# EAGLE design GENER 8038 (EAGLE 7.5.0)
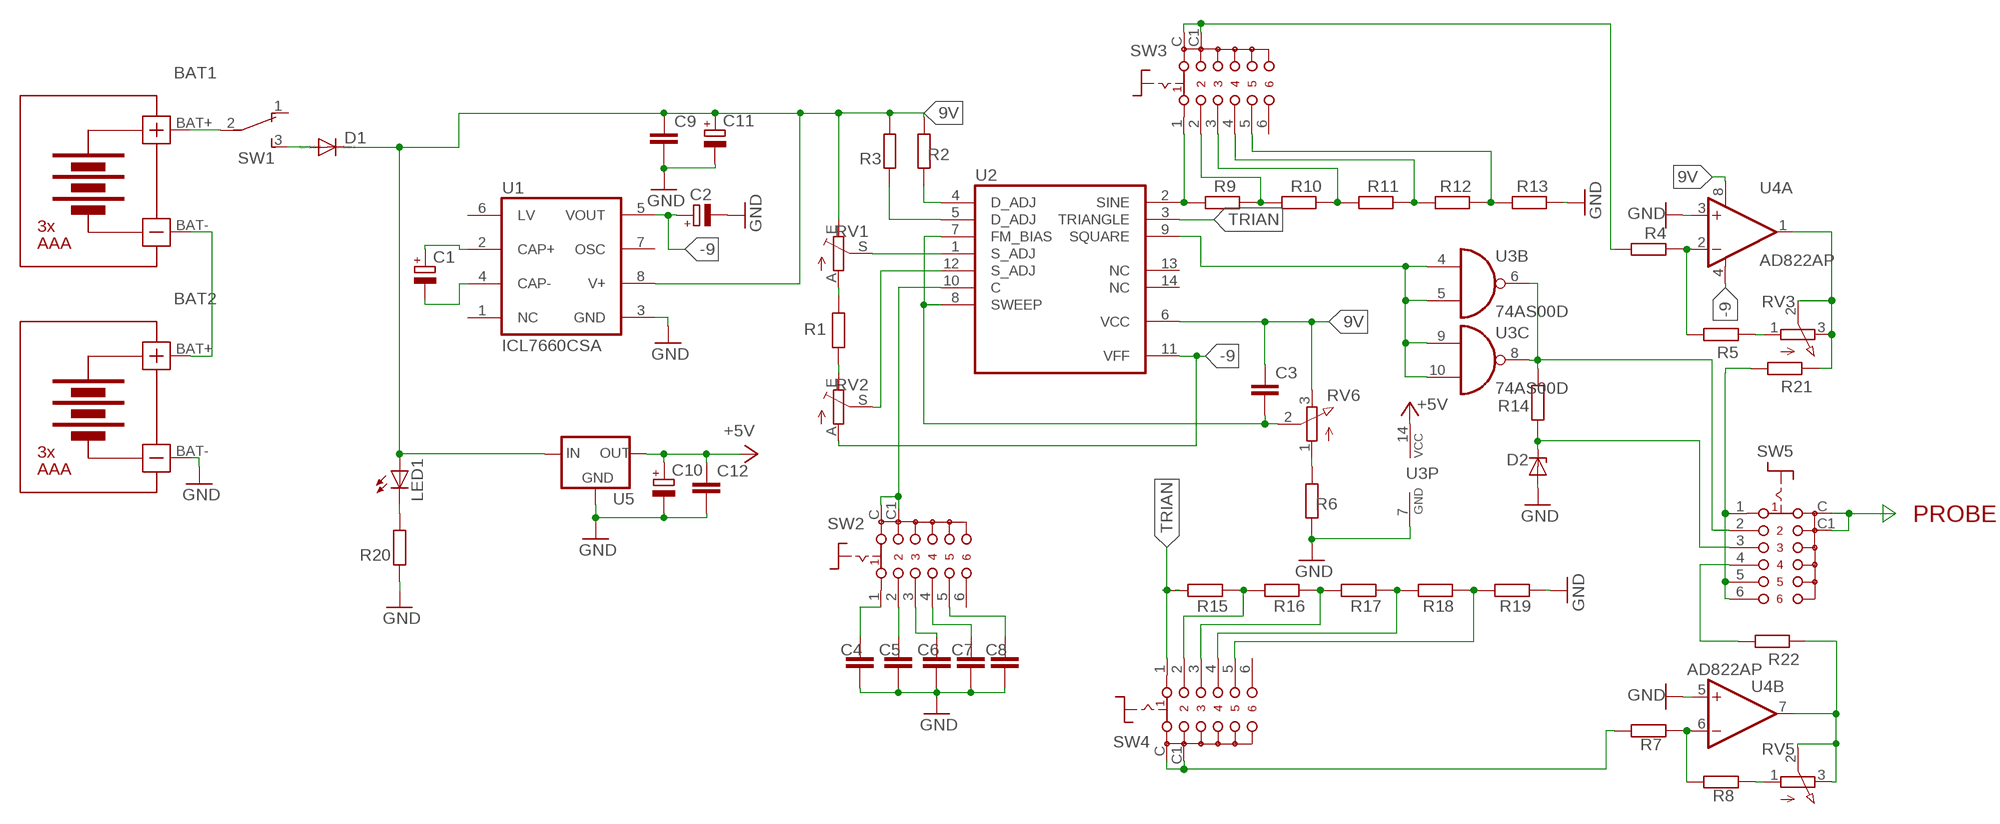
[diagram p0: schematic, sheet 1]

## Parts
BAT1  BATTERY-HOLDER-3AAA  [BATTERY-HOLDER-3AAA]
BAT2  BATTERY-HOLDER-3AAA  [BATTERY-HOLDER-3AAA]
C1  CPOL-EUC/6032-28W  [C/6032-28W]
C2  CPOL-EUC/6032-28W  [C/6032-28W]
C3  C-EUC1206  [C1206]
C4  C-EUC1206  [C1206]
C5  C-EUC1206  [C1206]
C6  C-EUC1206  [C1206]
C7  C-EUC1206  [C1206]
C8  C-EUC1206  [C1206]
C9  C-EUC1206  [C1206]
C10  CPOL-EUC/6032-28W  [C/6032-28W]
C11  CPOL-EUC/6032-28W  [C/6032-28W]
C12  C-EUC1206  [C1206]
D1  1N4148DO35-7  [DO35-7]
D2  BZX85  [DO41Z10]
LED1  LED3MM  [LED3MM]
R1  R-EU_R1206  [R1206]
R2  R-EU_R1206  [R1206]
R3  R-EU_R1206  [R1206]
R4  R-EU_R1206  [R1206]
R5  R-EU_R1206  [R1206]
R6  R-EU_R1206  [R1206]
R7  R-EU_R1206  [R1206]
R8  R-EU_R1206  [R1206]
R9  R-EU_R1206  [R1206]
R10  R-EU_R1206  [R1206]
R11  R-EU_R1206  [R1206]
R12  R-EU_R1206  [R1206]
R13  R-EU_R1206  [R1206]
R14  R-EU_R1206  [R1206]
R15  R-EU_R1206  [R1206]
R16  R-EU_R1206  [R1206]
R17  R-EU_R1206  [R1206]
R18  R-EU_R1206  [R1206]
R19  R-EU_R1206  [R1206]
R20  R-EU_R1206  [R1206]
R21  R-EU_R1206  [R1206]
R22  R-EU_R1206  [R1206]
RV1  TRIM_EU-CT6  [CT6]
RV2  TRIM_EU-CT6  [CT6]
RV3  PTV09A  PV09A  [PTV09]
RV5  PTV09A  PV09A  [PTV09]
RV6  PTV09A  PV09A  [PTV09]
SW1  TL36YO  [TL3XYO]
SW2  SS-10-16  [SS-10-16]
SW3  SS-10-16  [SS-10-16]
SW4  SS-10-16  [SS-10-16]
SW5  SS-10-16  [SS-10-16]
U1  ICL7660CSA  [SO08]
U2  XR-8038  [DIL14]
U3  74AS00D  [SO14]
U4  AD822AP  OPA2131U  [SO08]
U5  78LXX  [78LXX]

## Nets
9V: C3.1 C9.1 C11.+ D1.C LED1.A R2.2 R3.2 RV1.E RV6.3(E) U1.8(V+) U2.6(VCC) U4.8(A:V+) U5.IN
+5V: C10.+ C12.1 U3.14(P:VCC) U5.OUT
-9: C2.+ RV2.A U1.5(VOUT) U2.11(VFF) U4.4(A:V-)
GND: BAT2.BAT- C2.- C4.2 C5.2 C6.2 C7.2 C8.2 C9.2 C10.- C11.- C12.2 D2.A R6.1 R13.1 R19.1 R20.1 U1.3(GND) U3.7(P:GND) U4.3(A:+IN) U4.5(B:+IN) U5.GND
N$1: BAT1.BAT- BAT2.BAT+
N$2: BAT1.BAT+ SW1.2(P)
N$3: R2.1 U2.4(D_ADJ)
N$4: R3.1 U2.5(D_ADJ)
N$5: RV1.S U2.1(S_ADJ)
N$6: R1.2 RV1.A
N$7: R1.1 RV2.E
N$8: RV2.S U2.12(S_ADJ)
N$9: C3.2 RV6.2(S) U2.7(FM_BIAS) U2.8(SWEEP)
N$10: SW2.C SW2.C1 U2.10(C)
N$11: R6.2 RV6.1(A)
N$12: C4.1 SW2.1
N$13: C5.1 SW2.2
N$14: C6.1 SW2.3
N$15: C7.1 SW2.4
N$16: C8.1 SW2.5
N$17: R9.2 SW3.1 U2.2(SINE)
N$18: R9.1 R10.2 SW3.2
N$19: R10.1 R11.2 SW3.3
N$20: R11.1 R12.2 SW3.4
N$21: R12.1 R13.2 SW3.5
N$22: U2.9(SQUARE) U3.4(B:I0) U3.5(B:I1) U3.9(C:I0) U3.10(C:I1)
N$23: R15.1 R16.2 SW4.2
N$24: R16.1 R17.2 SW4.3
N$25: R17.1 R18.2 SW4.4
N$26: R18.1 R19.2 SW4.5
N$27: R14.2 SW5.2 U3.6(B:O) U3.8(C:O)
N$28: D2.C R14.1 SW5.3
N$29: R21.2 SW5.1 SW5.5 SW5.6
N$30: R4.1 R5.2 U4.2(A:-IN)
N$31: R5.1 RV3.1(A)
N$32: R4.2 SW3.C SW3.C1
N$33: R7.1 R8.2 U4.6(B:-IN)
N$34: R8.1 RV5.1(A)
N$35: R22.1 RV5.2(S) RV5.3(E) U4.7(B:OUT)
N$36: R7.2 SW4.C SW4.C1
N$37: SW5.C SW5.C1
N$38: D1.A SW1.3(S)
N$39: LED1.K(C) R20.2
N$40: R21.1 RV3.2(S) RV3.3(E) U4.1(A:OUT)
N$41: R22.2 SW5.4
N$84: C1.+ U1.2(CAP+)
N$85: C1.- U1.4(CAP-)
TRIAN: R15.2 SW4.1 U2.3(TRIANGLE)
Unconnected: SW1.1(O) SW2.6 SW3.6 SW4.6 U1.1(NC) U1.6(LV) U1.7(OSC) U2.13(NC) U2.14(NC) U3.1(A:I0) U3.2(A:I1) U3.3(A:O) U3.11(D:O) U3.12(D:I0) U3.13(D:I1)

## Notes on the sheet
- PROBE

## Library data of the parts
BAT1 BAT2 = diy-modules:BATTERY-HOLDER-3AAA
C1 C2 C10 C11 = rcl:CPOL-EU: POLARIZED CAPACITOR, European symbol
C3-C9 C12 = rcl:C-EU: CAPACITOR, European symbol
D1 = diode:1N4148: DIODE
D2 = diode:BZX85: Z DIODE
LED1 = led:LED: LED
R1-R22 = rcl:R-EU_: RESISTOR, European symbol
RV1 RV2 = pot:TRIM_EU-: POTENTIOMETER
RV3 RV5 RV6 = pot:PV09A
SW1 = switch:TL36YO: TINY SWITCH ON - ON Source: http://www2.produktinfo.conrad.com/datenblaetter/700000-724999/705152-da-01-de-Subminiaturschalter_TL_36YO.pdf
SW2-SW5 = switch:SS-10-16: Rotary Switch, Through Hole, 6 Position, 1 Pole
U1 = maxim:ICL7660CSA: VOLTAGE CONVERTER; MF: MAXIM; MPN: ICL7660CSA; OC_FARNELL: 9724710; OC_NEWARK: 34C3732
U2 = exar:XR-8038: Precision WAVEFORM GENERATOR; OC_FARNELL: unknown; OC_NEWARK: unknown
U3 = 74xx-eu:74*00: Quad 2-input NAND gate
U4 = burr-brown:OPA2131: General Purpose FET-Input Operational Amplifiers Product Folder:OPA2131; MF: TEXAS INSTRUMENT CONNECTORS; MPN: OPA2131UJ/2K5; OC_FARNELL: 1575488; OC_NEWARK: 75C4620
U5 = v-reg:78LXX: VOLTAGE REGULATOR

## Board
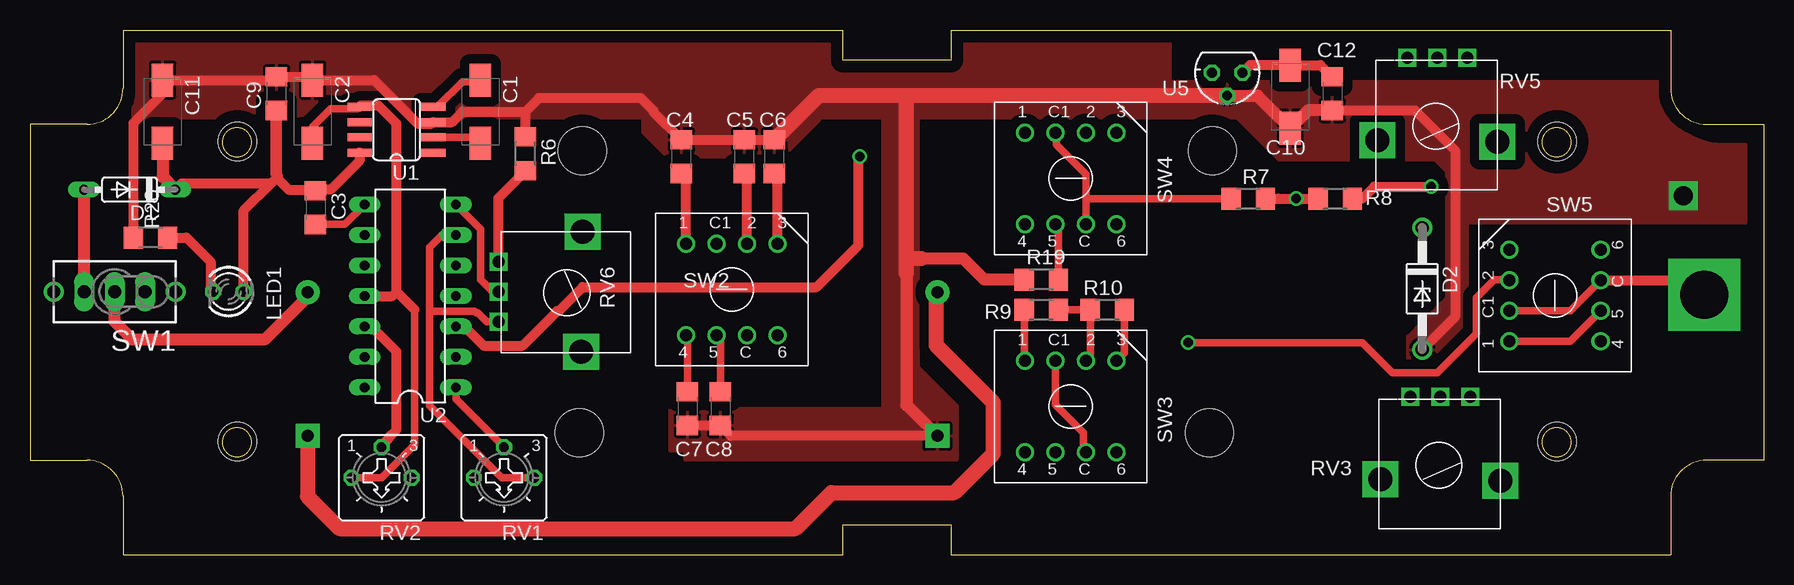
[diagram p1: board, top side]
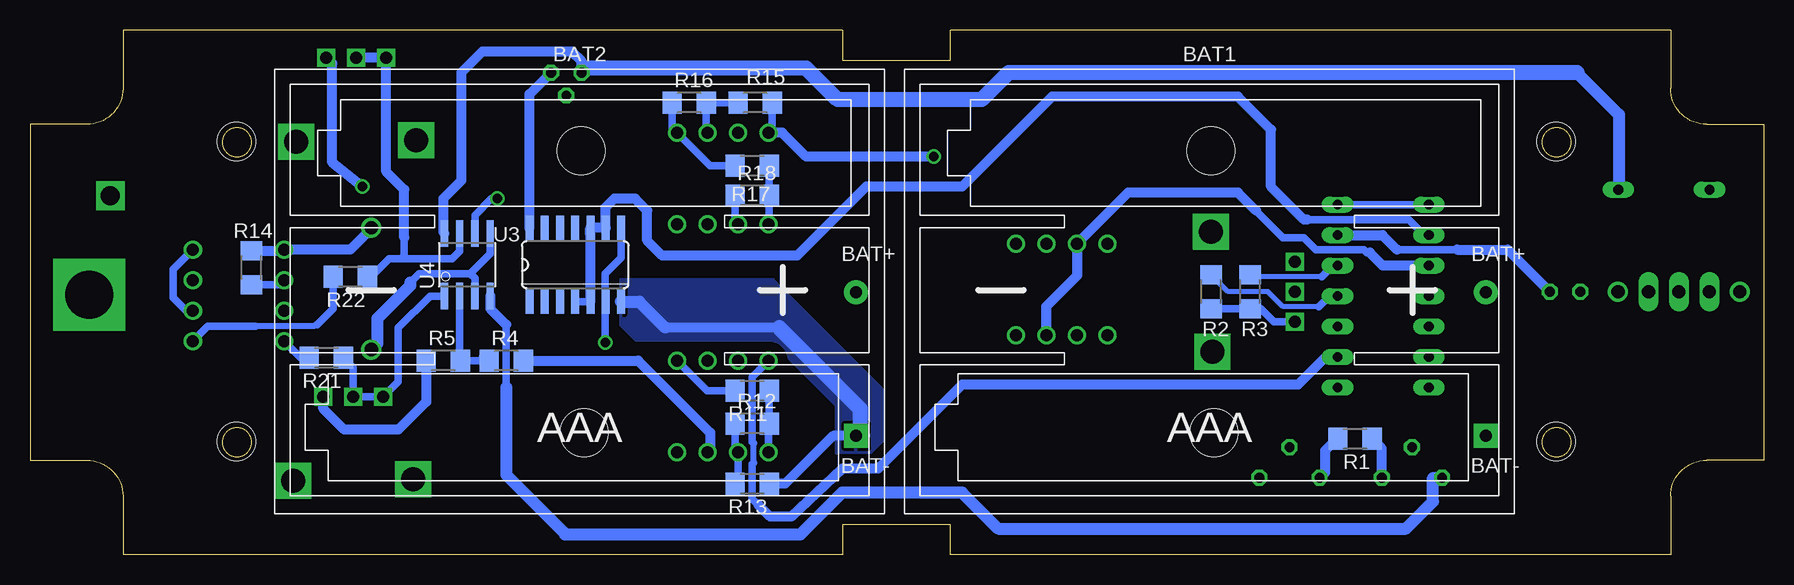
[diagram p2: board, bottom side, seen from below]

Size 144.5 x 43.72 mm. Coordinates in mm from the lower left corner, seen from the top.
Outline: 76.75,41.22 67.75,41.22 67.75,43.72 7.75,43.72 7.75,38.86 arc-90 4.75,35.86 0,35.86 0,7.86 4.75,7.86 arc-90 7.75,4.86 7.75,0 67.75,0 67.75,2.5 76.75,2.5 76.75,0 136.75,0 136.75,4.86 arc-90 139.75,7.86 144.5,7.86 144.5,35.86 139.75,35.86 arc-90 136.75,38.86 136.75,43.72 76.75,43.72 76.75,41.22
Outline: circle at 17.25,34.36 radius 1.2
Outline: circle at 17.25,9.36 radius 1.2
Outline: circle at 127.25,34.36 radius 1.2
Outline: circle at 127.25,9.36 radius 1.2
Copper layers (1*16): Top 0.035mm / dielectric 1.5mm / Bottom 0.035mm
Design rules "default": minimum track width 10mil, minimum drill 24mil, track to track 8mil, track to pad 8mil, pad to pad 8mil, via to via 8mil, smd to smd 8mil, copper to edge 40mil, drill to drill 8mil, minimum pad ring 10mil, minimum via ring 8mil, stop-mask expansion 4mil, vias tented up to drill 0mil, thermal gap 10mil
Holes 3.2 mm at 17.3,34.41 17.3,9.41 127.3,34.41 127.3,9.41

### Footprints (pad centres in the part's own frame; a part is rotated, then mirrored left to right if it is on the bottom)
BATTERY-HOLDER-3AAA = drill 1 pad 2: BAT+ 22.425,0.46 | drill 1 pad 2 square: BAT- 22.425,-11.51 | hole 4: -0.5,12.25; -0.25,-11.25
C/6032-28W = smd 2.75 x 1.8: + 2.625,0; - -2.625,0
C1206 = smd 1.6 x 1.8: 1 -1.4,0; 2 1.4,0
DO35-7 = drill 0.813 long: A 3.81,0; C -3.81,0
DO41Z10 = drill 1.118: A 5.08,0; C -5.08,0
LED3MM = drill 0.813 octagon: A -1.27,0; K 1.27,0
R1206 = smd 1.6 x 1.803: 1 -1.422,0; 2 1.422,0
CT6 = drill 0.813 octagon: A 2.515,0; E -2.515,0; S 0,-2.54
PTV09 = drill 1 square: 1 -2.5,0; 2 0,0; 3 2.5,0 | drill 2 square: P$4 -5,7; P$5 5,6.9
TL3XYO = drill 1.1 pad 1.422 long: 1 -2.54,0; 2 0,0; 3 2.54,0 | drill 1.1 pad 1.676: M1 -5.08,0; M2 5.08,0
SS-10-16 = drill 1: 1 -7.62,0; 2 -2.54,0; 3 0,0; 4 -7.62,-7.62; 5 -5.08,-7.62; 6 0,-7.62; C -2.54,-7.62; C1 -5.08,0
SO08 = smd 0.66 x 2.032: 1 -1.905,-3.073; 2 -0.635,-3.073; 3 0.635,-3.073; 4 1.905,-3.073; 5 1.905,3.073; 6 0.635,3.073; 7 -0.635,3.073; 8 -1.905,3.073
DIL14 = drill 0.813 long: 1 -7.62,-3.81; 2 -5.08,-3.81; 3 -2.54,-3.81; 4 0,-3.81; 5 2.54,-3.81; 6 5.08,-3.81; 7 7.62,-3.81; 8 7.62,3.81; 9 5.08,3.81; 10 2.54,3.81; 11 0,3.81; 12 -2.54,3.81; 13 -5.08,3.81; 14 -7.62,3.81
SO14 = smd 0.66 x 2.032: 1 -3.81,-3.073; 2 -2.54,-3.073; 3 -1.27,-3.073; 4 0,-3.073; 5 1.27,-3.073; 6 2.54,-3.073; 7 3.81,-3.073; 8 3.81,3.073; 9 2.54,3.073; 10 1.27,3.073; 11 0,3.073; 12 -1.27,3.073; 13 -2.54,3.073; 14 -3.81,3.073
SO08' = smd 0.61 x 2.21: 1 -1.905,-2.616; 2 -0.635,-2.616; 3 0.635,-2.616; 4 1.905,-2.616; 5 1.905,2.616; 6 0.635,2.616; 7 -0.635,2.616; 8 -1.905,2.616
78LXX = drill 0.813 octagon: GND 0,1.905; IN 1.27,0; OUT -1.27,0

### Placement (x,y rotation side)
BAT1  45.55,21.41 0 bottom
BAT2  98.05,21.41 0 bottom
C1  37.55,36.91 270 top
C2  23.55,36.91 270 top
C3  23.8,28.91 270 top
C4  54.3,33.16 90 top
C5  59.55,33.16 90 top
C6  62.05,33.16 90 top
C7  54.8,12.16 270 top
C8  57.55,12.16 270 top
C9  20.55,38.41 90 top
C10  105.05,38.16 90 top
C11  11.05,36.91 270 top
C12  108.55,38.41 270 top
D1  8.3,30.41 180 top
D2  116.05,22.16 270 top
LED1  16.55,21.91 180 top
R1  34.05,9.66 180 bottom
R2  46.05,21.91 270 bottom
R3  42.8,21.91 270 bottom
R4  104.8,16.16 0 bottom
R5  110.05,16.16 0 bottom
R6  41.3,33.41 270 top
R7  101.55,29.66 180 top
R8  108.8,29.66 180 top
R9  84.3,20.41 180 top
R10  89.8,20.41 180 top
R11  84.3,13.66 180 bottom
R12  84.3,10.91 0 bottom
R13  84.3,5.91 180 bottom
R14  126.05,23.91 270 bottom
R15  84.05,37.66 0 bottom
R16  89.55,37.66 0 bottom
R17  84.3,32.41 180 bottom
R18  84.3,29.91 0 bottom
R19  84.3,22.91 0 top
R20  10.05,26.41 0 top
R21  119.8,16.41 180 bottom
R22  117.8,23.16 180 bottom
RV1  39.51,6.41 180 top
RV2  29.3,6.41 180 top
RV3  117.55,13.16 180 top
RV5  117.3,41.41 180 top
RV6  39.05,21.91 270 top
SW1  7.05,21.91 180 top
SW2  62.3,25.91 0 top
SW3  90.55,16.16 0 top
SW4  90.55,35.16 0 top
SW5  123.3,25.41 90 top
U1  30.55,35.41 90 top
U2  31.7,21.55 90 top
U3  99.05,24.16 0 bottom
U4  AD822AP  [SO08']  108.05,24.16 0 bottom
U5  99.8,40.16 180 top

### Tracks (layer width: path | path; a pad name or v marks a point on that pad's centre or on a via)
9V
  Top 0.61: RV6.3 38.05,19.41 37.3,20.16 37.17,20.16 37.05,20.28 33.42,20.28 33.3,20.41 | U2.6 34.3,26.63 33.3,25.63 33.3,20.41 | 33.3,20.41 33.3,12.41 39.3,6.41 RV1.E
  Top 0.813: 20.55,31.41 C9.1 20.45,36.91 20.45,31.76 20.68,31.53 20.55,31.41 | 20.55,31.41 21.55,30.41 23.7,30.41 C3.1 23.9,30.41 25.05,30.41 27.48,32.83 U1.8 | LED1.A 17.82,28.68 20.05,30.91 | 20.05,30.91 20.55,31.41 | 20.05,30.91 12.61,30.91 D1.C
  Top 1.016: C11.+ 11.05,31.47 D1.C
  Bottom 0.61: 30.55,25.41 25.55,25.41 | RV6.3 40.8,19.41 41.88,20.49 R3.2 R2.2
  Bottom 0.813: U2.6 31.77,26.63 30.55,25.41 | 25.55,25.41 21.32,25.41 LED1.A | U5.IN 98.53,41.14 99.3,41.91 106.8,41.91 108.55,40.16 108.55,31.16 110.05,29.66 110.05,26.87 U4.8
  Bottom 1.016: 15.55,40.16 12.05,36.66 12.05,30.47 D1.C
  Bottom 1.27: 15.55,40.16 62.92,40.16 65.17,37.91 77.17,37.91 79.8,40.53 98.16,40.53 U5.IN
+5V
  Top 0.813: U5.OUT 101.69,40.78 C10.+ 107.58,40.78 C12.1
  Bottom 0.813: U3.14 102.86,38.37 U5.OUT
-9
  Top 0.61: C2.+ 23.55,35.66 25.05,37.16 27.32,37.16 U1.5 | 32.05,20.41 32.05,9.16 29.3,6.41 RV2.A
  Top 0.813: U2.11 30.19,21.55 30.55,21.91 | 30.55,21.91 30.55,35.91 29.05,37.41 27.57,37.41 U1.5 | 30.55,21.91 32.05,20.41
  Bottom 0.61: 104.8,19.16 104.8,13.91
  Bottom 0.813: U4.4 106.14,20.5 104.8,19.16
  Bottom 1.016: 104.8,13.91 104.8,6.66 99.94,1.79 99.94,1.66 80.3,1.66 76.8,5.16 66.8,5.16 63.8,2.16 29.8,2.16 27.55,4.41 27.55,6.39 RV2.A
GND  (via drill 1.6)
  Top 0.813: 41.3,36.91 36.05,36.91 35.19,36.04 U1.3 33.49,35.91 32.3,35.91 28.68,39.53 C2.- 23.27,39.81 C9.2 20.27,39.53 C11.- 10.93,39.41 10.93,38.28 8.63,35.99 R20.1 | C6.2 C5.2 C4.2 51.95,36.91 51.95,37.01 50.92,38.03 42.42,38.03 41.3,36.91 | R6.1 41.3,36.91 | C7.2 C8.2 58.41,9.9 BAT2.BAT- | C12.2 115.45,37.01 118.8,33.66 118.8,19.83 D2.A
  Top 1.016: R19.1 79.55,22.91 77.8,24.66 74.3,24.66 | 73.05,23.41 73.05,12.47 BAT2.BAT- | U5.GND 102.33,38.25 C10.- 106.52,37.01 C12.2
  Top 1.27: U5.GND 72.8,38.25 | 72.8,38.25 65.75,38.25 C6.2 | 73.05,23.41 73.05,24.66 | 73.05,24.66 73.05,38 72.8,38.25 | 74.3,24.66 73.05,24.66
  Bottom 0.61: U4.3 107.41,23.02 107.8,23.41 | 107.8,23.41 112.05,23.41 112.8,22.66 | U4.5 106.14,25.06 107.8,23.41
  Bottom 0.813: 82.05,18.91 91.55,18.91 | BAT2.BAT- 77.56,9.9 81.55,5.91 R13.1
  Bottom 1.016: U3.7 93.73,21.08 91.55,18.91 | 112.8,22.66 112.8,22.41 115.55,19.66 115.55,17.58 D2.A
  Bottom 1.27: 82.05,18.91 75.3,12.16 75.3,10.22 BAT2.BAT-
  other vias: 137.8,29.91
  pour Top (isolate 0.813): 143.05,34.16 141.05,34.16 arc-90 135.8,39.41 95.05,39.41 95.05,43.41 77.55,43.41 77.55,40.66 67.05,40.66 67.05,43.16 66.8,43.16 8.55,43.16 8.55,36.41 71.05,36.41 71.05,12.16 53.3,12.16 53.3,8.66 54.55,8.66 54.55,7.91 77.3,7.91 77.3,12.41 74.05,15.66 74.05,36.41 100.55,36.41 104.05,32.91 117.05,32.91 118.05,31.91 118.05,21.41 115.55,18.91 114.8,18.16 114.8,15.91 116.3,15.91 119.8,19.41 119.8,27.66 143.05,27.66
  pour Bottom (isolate 0.813): 94.55,22.91 95.3,22.91 95.8,22.41 95.8,19.66 94.05,17.91 82.8,17.91 77.3,12.41 77.3,8.41 77.05,8.16 74.05,8.16 73.3,8.91 73.3,13.66 82.55,22.91
  pour Top (isolate 0.813): 51.05,36.66 51.05,35.16 53.05,33.16 62.8,33.16 65.8,36.16 65.8,39.16 51.3,39.16 51.05,39.16
N$1
  Top 1.27: BAT1.BAT- 23.12,4.83 25.8,2.16 63.8,2.16 66.8,5.16 77.05,5.16 80.3,8.41 80.3,12.66 75.55,17.41 75.55,21.79 BAT2.BAT+
N$2
  Top 1.016: BAT1.BAT+ 23.12,21.48 19.55,17.91 8.55,17.91 7.05,19.41 SW1.2
N$3
  Bottom 0.406: 37.05,20.66 40.05,20.66 41.3,21.91 44.63,21.91 R2.1
  Bottom 0.61: U2.4 36.16,21.55 37.05,20.66
N$4
  Bottom 0.406: 36.8,23.16 42.63,23.16
  Bottom 0.61: U2.5 35.87,24.09 36.8,23.16 | 42.63,23.16 R3.1
N$5
  Top 0.61: U2.1 35.51,12.95 RV1.S
N$6
  Bottom 0.813: R1.2 35.55,9.66 36.55,8.66 36.55,6.85 RV1.A
N$7
  Bottom 0.813: RV2.E 31.82,8.84 R1.1
N$8
  Top 0.813: RV2.S 30.05,9.91 30.55,10.41 30.55,16.91 28.55,18.91 27.99,18.91 U2.12
N$9
  Top 0.61: RV6.2 38.55,21.91 37.55,22.91 37.55,27.13 U2.7 | C3.2 26.23,27.51 U2.8
  Bottom 0.61: U2.7 U2.8
N$10
  Bottom 0.61: 32.8,25.16 33.05,25.16 33.3,25.41 37.3,25.41 38.3,26.41 40.05,26.41 42.3,28.66
  Bottom 0.813: U2.10 31.73,24.09 32.8,25.16 | SW2.C 59.8,18.33 59.8,20.66 57.22,23.24 SW2.C1 52.97,30.16 43.8,30.16 42.3,28.66
N$11
  Top 0.813: RV6.1 39.05,29.74 R6.2
N$12
  Top 0.813: SW2.1 54.68,31.38 C4.1
N$13
  Top 0.813: SW2.2 59.76,31.55 C5.1
N$14
  Top 0.813: SW2.3 62.3,31.51 C6.1
N$15
  Top 0.61: C7.1 54.8,18.17 SW2.4
N$16
  Top 0.61: C8.1 57.55,17.96 SW2.5
N$17
  Top 0.61: R9.2 82.88,16.21 SW3.1
  Bottom 0.5: 84.17,7.66 84.17,9.28
  Bottom 0.61: SW3.1 84.3,14.79 84.3,9.41 84.17,9.28 | 83.8,4.16 84.3,4.66 84.3,7.53 84.17,7.66
  Bottom 0.813: U2.2 36.49,16.47 38.8,14.16 66.8,14.16 73.8,7.16 76.8,7.16 81.05,3.16 82.8,3.16 83.8,4.16
N$18
  Top 0.61: SW3.2 88.38,16.53 R10.2 R9.1
N$19
  Top 0.61: R10.1 91.22,16.83 SW3.3
  Bottom 0.61: R11.2 88.05,13.66 SW3.3
N$20
  Bottom 0.61: SW3.4 82.93,10.86 R12.2 R11.1
N$21
  Bottom 0.61: R13.2 85.47,6.66 SW3.5 85.72,8.79 R12.1
N$22
  Bottom 0.61: U2.9 28.27,26.63 29.55,27.91 38.05,27.91 | U3.4 U3.5
  Bottom 0.813: U3.5 97.78,26.64 97.8,26.66 97.8,27.21 U3.10 U3.9 96.55,27.27 96.55,28.91 95.8,29.66 94.05,29.66 93.05,28.66 93.05,26.16 91.8,24.91 80.55,24.91 74.92,30.53 74.8,30.66 66.8,30.66 59.3,38.16 43.8,38.16 41.05,35.41 41.05,30.66 38.3,27.91 38.05,27.91
N$23
  Bottom 0.61: SW4.2 88.13,35.28 R16.2 R15.1
N$24
  Bottom 0.61: R17.2 87.8,32.41 SW4.3 90.97,35.58 R16.1
N$25
  Bottom 0.61: R17.1 R18.2 82.88,27.59 SW4.4
N$26
  Top 0.61: R19.2 85.72,27.29 SW4.5
  Bottom 0.61: R18.1 85.72,27.79 SW4.5
N$27  (via drill 0.8)
  Top 0.61: v96.55,17.66 111.05,17.66 113.55,15.16 117.3,15.16 120.55,18.41 120.55,21.41 122.05,22.91 123.26,22.91 SW5.2
  Bottom 0.61: U3.8 95.24,24.72 96.55,23.41 96.55,21.12 | 96.55,21.12 U3.6 | R14.2 123.68,22.49 SW5.2 | 96.55,21.12 v96.55,17.66
N$28
  Bottom 0.813: D2.C 116.05,27.16 117.8,25.41 122.8,25.41 | 122.8,25.41 SW5.3 | R14.1 122.88,25.33 122.8,25.41
N$29
  Top 0.61: SW5.1 128.38,17.79 SW5.5
  Bottom 0.61: SW5.5 131.47,20.33 132.55,21.41 132.55,23.78 SW5.6 | R21.2 121.92,16.41 SW5.1
N$30
  Bottom 0.61: U4.2 108.69,16.21 R5.2 106.8,16.16 106.8,16.41 106.47,16.41 R4.1
N$31
  Bottom 0.813: R5.1 111.47,12.74 113.8,10.41 118.3,10.41 120.05,12.16 RV3.1
N$32
  Top 0.61: SW3.C1 85.47,12.49 87.8,10.16 87.8,8.75 SW3.C
  Bottom 0.813: R4.2 93.8,16.16 87.8,10.16 87.8,8.75 SW3.C
N$33  (via drill 0.8)
  Top 0.813: R7.1 104.05,29.66 v105.55,29.66 R8.2
  Bottom 0.61: U4.6 107.41,28.29 106.05,29.66 v105.55,29.66
N$34  (via drill 0.8)
  Top 0.813: R8.1 111.05,29.66 112.05,30.66 v116.8,30.66
  Bottom 0.813: v116.8,30.66 119.3,32.66 119.3,40.91 RV5.1
N$35
  Bottom 0.61: U4.7 108.69,25.27 109.3,24.66 113.55,24.66 | R22.1 116.05,23.16 114.55,24.66 113.55,24.66 | 113.3,26.41 113.3,24.91 113.55,24.66
  Bottom 0.813: 113.3,26.41 113.3,30.41 114.8,31.91 RV5.3 RV5.2
N$36
  Top 0.61: SW4.C 88.01,29.41 | 88.01,29.41 88.01,31.7 85.55,34.16 85.55,35.08 SW4.C1 | R7.2 88.26,29.66 88.01,29.41
N$37  (via drill 4 pad 6)
  Top 0.61: SW5.C1 128.38,20.33 SW5.C
  Top 0.813: SW5.C 138.34,22.87 v139.55,21.66
N$38
  Top 1.016: D1.A 4.49,21.93 SW1.3
N$39
  Top 0.813: R20.2 13.05,26.41 15.05,24.41 15.05,22.14 LED1.K
N$40
  Bottom 0.61: U4.1 111.17,21.54 113.8,18.91 113.8,14.41 RV3.3 RV3.2 117.55,15.58 R21.1
N$41
  Bottom 0.5: 120.55,19.16 120.67,19.16 120.8,19.03 125.67,19.03
  Bottom 0.61: R22.2 119.22,20.49 120.55,19.16 | 125.67,19.03 129.68,19.03 SW5.4
N$84
  Top 0.61: U1.2 37.06,34.77 C1.+
N$85
  Top 0.61: U1.4 33.95,37.31 36.05,39.41 37.42,39.41 C1.-
TRIAN  (via drill 0.8)
  Top 0.813: U2.3 36.2,19.01 37.8,17.41 41.05,17.41 43.92,20.28 44.05,20.28 46.05,22.28 65.55,22.28 69.05,25.78 69.05,33.03 v69.17,33.16
  Bottom 0.61: R15.2 82.63,35.46 SW4.1
  Bottom 0.813: v69.17,33.16 79.8,33.16 81.8,35.16 SW4.1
